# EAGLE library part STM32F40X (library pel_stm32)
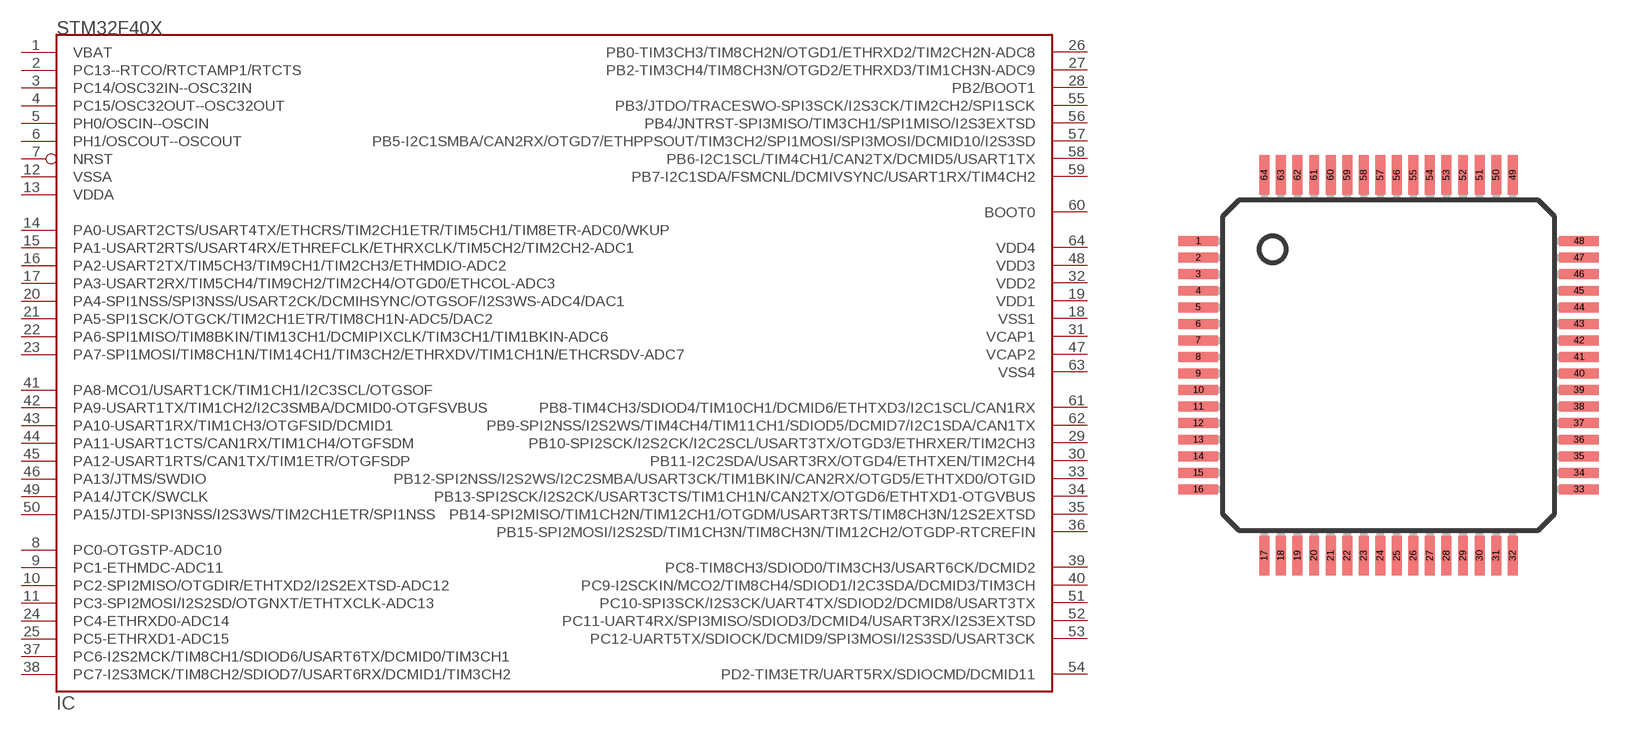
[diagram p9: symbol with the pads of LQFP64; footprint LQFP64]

Designator prefix IC

## STM32F40X  [LQFP64]
1  VBAT  sup
2  PC13--RTCO/RTCTAMP1/RTCTS
3  PC14/OSC32IN--OSC32IN
4  PC15/OSC32OUT--OSC32OUT
5  PH0/OSCIN--OSCIN  in
6  PH1/OSCOUT--OSCOUT  out
7  NRST
8  PC0-OTGSTP-ADC10
9  PC1-ETHMDC-ADC11
10  PC2-SPI2MISO/OTGDIR/ETHTXD2/I2S2EXTSD-ADC12
11  PC3-SPI2MOSI/I2S2SD/OTGNXT/ETHTXCLK-ADC13
12  VSSA  sup
13  VDDA  sup
14  PA0-USART2CTS/USART4TX/ETHCRS/TIM2CH1ETR/TIM5CH1/TIM8ETR-ADC0/WKUP
15  PA1-USART2RTS/USART4RX/ETHREFCLK/ETHRXCLK/TIM5CH2/TIM2CH2-ADC1
16  PA2-USART2TX/TIM5CH3/TIM9CH1/TIM2CH3/ETHMDIO-ADC2
17  PA3-USART2RX/TIM5CH4/TIM9CH2/TIM2CH4/OTGD0/ETHCOL-ADC3
18  VSS1  sup
19  VDD1  sup
20  PA4-SPI1NSS/SPI3NSS/USART2CK/DCMIHSYNC/OTGSOF/I2S3WS-ADC4/DAC1
21  PA5-SPI1SCK/OTGCK/TIM2CH1ETR/TIM8CH1N-ADC5/DAC2
22  PA6-SPI1MISO/TIM8BKIN/TIM13CH1/DCMIPIXCLK/TIM3CH1/TIM1BKIN-ADC6
23  PA7-SPI1MOSI/TIM8CH1N/TIM14CH1/TIM3CH2/ETHRXDV/TIM1CH1N/ETHCRSDV-ADC7
24  PC4-ETHRXD0-ADC14
25  PC5-ETHRXD1-ADC15
26  PB0-TIM3CH3/TIM8CH2N/OTGD1/ETHRXD2/TIM2CH2N-ADC8
27  PB2-TIM3CH4/TIM8CH3N/OTGD2/ETHRXD3/TIM1CH3N-ADC9
28  PB2/BOOT1
29  PB10-SPI2SCK/I2S2CK/I2C2SCL/USART3TX/OTGD3/ETHRXER/TIM2CH3
30  PB11-I2C2SDA/USART3RX/OTGD4/ETHTXEN/TIM2CH4
31  VCAP1  sup
32  VDD2  sup
33  PB12-SPI2NSS/I2S2WS/I2C2SMBA/USART3CK/TIM1BKIN/CAN2RX/OTGD5/ETHTXD0/OTGID
34  PB13-SPI2SCK/I2S2CK/USART3CTS/TIM1CH1N/CAN2TX/OTGD6/ETHTXD1-OTGVBUS
35  PB14-SPI2MISO/TIM1CH2N/TIM12CH1/OTGDM/USART3RTS/TIM8CH3N/12S2EXTSD
36  PB15-SPI2MOSI/I2S2SD/TIM1CH3N/TIM8CH3N/TIM12CH2/OTGDP-RTCREFIN
37  PC6-I2S2MCK/TIM8CH1/SDIOD6/USART6TX/DCMID0/TIM3CH1
38  PC7-I2S3MCK/TIM8CH2/SDIOD7/USART6RX/DCMID1/TIM3CH2
39  PC8-TIM8CH3/SDIOD0/TIM3CH3/USART6CK/DCMID2
40  PC9-I2SCKIN/MCO2/TIM8CH4/SDIOD1/I2C3SDA/DCMID3/TIM3CH
41  PA8-MCO1/USART1CK/TIM1CH1/I2C3SCL/OTGSOF
42  PA9-USART1TX/TIM1CH2/I2C3SMBA/DCMID0-OTGFSVBUS
43  PA10-USART1RX/TIM1CH3/OTGFSID/DCMID1
44  PA11-USART1CTS/CAN1RX/TIM1CH4/OTGFSDM
45  PA12-USART1RTS/CAN1TX/TIM1ETR/OTGFSDP
46  PA13/JTMS/SWDIO
47  VCAP2  sup
48  VDD3  sup
49  PA14/JTCK/SWCLK
50  PA15/JTDI-SPI3NSS/I2S3WS/TIM2CH1ETR/SPI1NSS
51  PC10-SPI3SCK/I2S3CK/UART4TX/SDIOD2/DCMID8/USART3TX
52  PC11-UART4RX/SPI3MISO/SDIOD3/DCMID4/USART3RX/I2S3EXTSD
53  PC12-UART5TX/SDIOCK/DCMID9/SPI3MOSI/I2S3SD/USART3CK
54  PD2-TIM3ETR/UART5RX/SDIOCMD/DCMID11
55  PB3/JTDO/TRACESWO-SPI3SCK/I2S3CK/TIM2CH2/SPI1SCK
56  PB4/JNTRST-SPI3MISO/TIM3CH1/SPI1MISO/I2S3EXTSD
57  PB5-I2C1SMBA/CAN2RX/OTGD7/ETHPPSOUT/TIM3CH2/SPI1MOSI/SPI3MOSI/DCMID10/I2S3SD
58  PB6-I2C1SCL/TIM4CH1/CAN2TX/DCMID5/USART1TX
59  PB7-I2C1SDA/FSMCNL/DCMIVSYNC/USART1RX/TIM4CH2
60  BOOT0  in
61  PB8-TIM4CH3/SDIOD4/TIM10CH1/DCMID6/ETHTXD3/I2C1SCL/CAN1RX
62  PB9-SPI2NSS/I2S2WS/TIM4CH4/TIM11CH1/SDIOD5/DCMID7/I2C1SDA/CAN1TX
63  VSS4
64  VDD4

## Footprint LQFP64 (pad centres in mm)
Based on STM PCB landpattern recomendation
smd 1.2 x 0.3: 1 -5.75,3.75; 2 -5.75,3.25; 3 -5.75,2.75; 4 -5.75,2.25; 5 -5.75,1.75; 6 -5.75,1.25; 7 -5.75,0.75; 8 -5.75,0.25; 9 -5.75,-0.25; 10 -5.75,-0.75; 11 -5.75,-1.25; 12 -5.75,-1.75; 13 -5.75,-2.25; 14 -5.75,-2.75; 15 -5.75,-3.25; 16 -5.75,-3.75; 33 5.75,-3.75; 34 5.75,-3.25; 35 5.75,-2.75; 36 5.75,-2.25; 37 5.75,-1.75; 38 5.75,-1.25; 39 5.75,-0.75; 40 5.75,-0.25; 41 5.75,0.25; 42 5.75,0.75; 43 5.75,1.25; 44 5.75,1.75; 45 5.75,2.25; 46 5.75,2.75; 47 5.75,3.25; 48 5.75,3.75
smd 0.3 x 1.2: 17 -3.75,-5.75; 18 -3.25,-5.75; 19 -2.75,-5.75; 20 -2.25,-5.75; 21 -1.75,-5.75; 22 -1.25,-5.75; 23 -0.75,-5.75; 24 -0.25,-5.75; 25 0.25,-5.75; 26 0.75,-5.75; 27 1.25,-5.75; 28 1.75,-5.75; 29 2.25,-5.75; 30 2.75,-5.75; 31 3.25,-5.75; 32 3.75,-5.75; 49 3.75,5.75; 50 3.25,5.75; 51 2.75,5.75; 52 2.25,5.75; 53 1.75,5.75; 54 1.25,5.75; 55 0.75,5.75; 56 0.25,5.75; 57 -0.25,5.75; 58 -0.75,5.75; 59 -1.25,5.75; 60 -1.75,5.75; 61 -2.25,5.75; 62 -2.75,5.75; 63 -3.25,5.75; 64 -3.75,5.75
